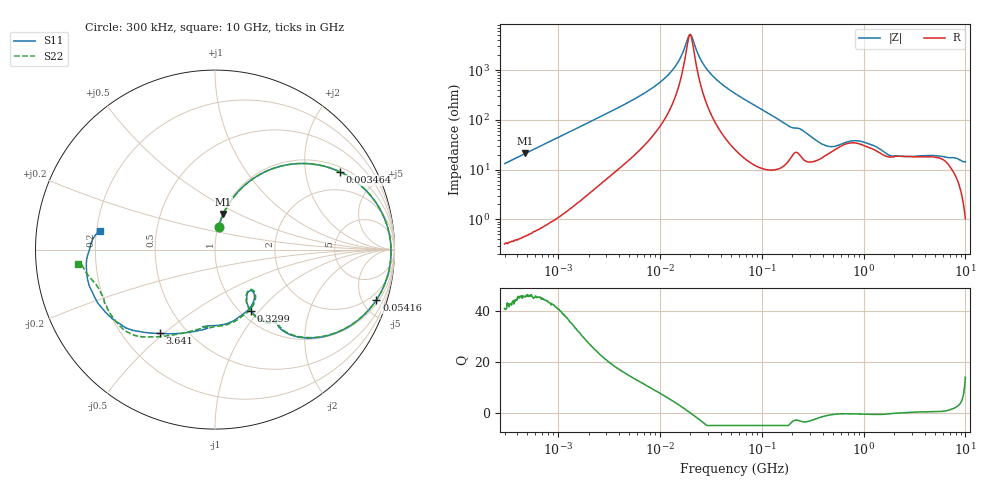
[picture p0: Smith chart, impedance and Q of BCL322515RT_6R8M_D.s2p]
! S-Parameter Data Generated by TDK Corporation
! Copyright(C) 2024 TDK Corporation.
! All Rights Reserved.
! TDK P/N: BCL322515RT-6R8M-D (SMD / SMT Inductor (Coil))
! Property: L=6.8uH at 1MHz
! Size(LxWxT): 3.2x2.5x1.5mm
! Model Type: s2p (Touchstone File Format Version 1.0)
! Frequency: DC=Yes Start=0.3MHz Stop=10000MHz 802points Log-sweep
! Model Generated on May 28, 2024
! Terms and conditions regarding TDK Simulation Models:
! 1)This simulation model is being provided solely for informational
!  purposes. Please refer to the specifications of the products in
!  terms of detailed characteristics of such products.
! 2)In no event shall TDK Corporation of any of its subsidiaries be
!  liable for any loss or damage arising, directly or indirectly,
!  from any information contained in this simulation model, including,
!  but not limited to loss or damages arising from any inaccuracies,
!  omissions or errors in connection with such information.
! 3)Any and all copyrights on this simulation model are owned by
!  TDK Corporation.  Duplication or redistribution of this simulation
!  model without prior written permission from TDK Corporation
!  is prohibited.
! 4)This simulation model is subject to any modification or change
!  without any prior notice.
! 5)Neither TDK Corporation nor any of its subsidiaries shall make any
!  warranty, express or implied, including but not limited to the
!  correctness, implied warranties of merchantability and fitness for
!  a particular purpose with respect to this simulation models.
! 6)The use of this simulation model shall be deemed to have consented
!  to the terms and conditions hereof.
! Port Assignments:
!  1 ---@@@--- 2
! Applicable Conditions:
!  Temperature = 25 degC
!  DC Bias Current = 0 A
!  Small Signal Operation
# Hz S MA R 50
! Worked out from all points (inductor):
!   801 points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, 300 kHz to 10 GHz, reference 50 ohm
!   read as one part in series: L = 7.02 uH near 318.3 kHz
!   highest Q = 45.8 at 478.9 kHz (marker M1), where L = 7.02 uH
!   self-resonance near 19.85 MHz
!   S11 on the Smith chart (normalised r, x): 300 kHz: 1.01, +0.26; 3.464 MHz: 1.17, +3.10; 54.16 MHz: 1.26, -6.30; 329.9 MHz: 1.12, -0.91; 3.641 GHz: 0.36, -0.48; 10 GHz: 0.21, +0.08
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300000  0.1287 80.9  0.9884 -7.6  0.9884 -7.6  0.1289 81.0
478871  0.2044 76.7  0.9741 -12.0  0.9744 -11.9  0.2045 76.8
942458  0.3805 66.2  0.9153 -22.5  0.9158 -22.4  0.3805 66.2
1713600  0.594 51.6  0.7848 -36.5  0.7851 -36.5  0.594 51.6
3464350  0.8199 31.8  0.5302 -55.1  0.5304 -55.1  0.82 31.9
9671944  0.9615 10.0  0.1803 -72.9  0.1803 -72.9  0.9616 10.0
1.421446e7  0.9766 4.1  0.08207 -71.6  0.08208 -71.6  0.9768 4.2
1.990974e7  0.9811 -0.6  0.01891 1.6  0.01892 1.7  0.9811 -0.6
2.856806e7  0.9777 -5.9  0.09003 72.4  0.09007 72.4  0.9778 -5.9
5.416364e7  0.9418 -17.4  0.2728 68.4  0.2729 68.4  0.9419 -17.3
5.477226e7  0.9407 -17.6  0.2765 68.2  0.2766 68.2  0.9408 -17.5
1.323997e8  0.7356 -42.0  0.6186 43.4  0.6188 43.4  0.7361 -41.7
1.855783e8  0.5673 -50.4  0.7188 28.7  0.719 28.7  0.5725 -49.9
3.126428e8  0.4183 -59.0  0.8 14.7  0.8003 14.7  0.4176 -59.5
3.29906e8  0.3965 -59.5  0.8061 12.7  0.8063 12.7  0.3953 -60.0
5.911415e8  0.3094 -48.3  0.7518 -4.3  0.7521 -4.3  0.3039 -47.3
9.101824e8  0.3786 -59.0  0.7083 -8.0  0.7085 -8.1  0.3812 -57.2
1.767019e9  0.4246 -93.3  0.7507 -23.2  0.7509 -23.3  0.4284 -90.2
3.640519e9  0.5594 -123.5  0.6338 -53.4  0.634 -53.5  0.5584 -120.4
6.495326e9  0.6921 -147.0  0.4956 -78.5  0.4957 -78.7  0.6823 -145.4
8.211115e9  0.7272 -168.9  0.4392 -98.1  0.4398 -98.2  0.695 -164.4
1e10  0.6503 171.0  0.3449 -110.6  0.3447 -110.8  0.7672 -173.8
